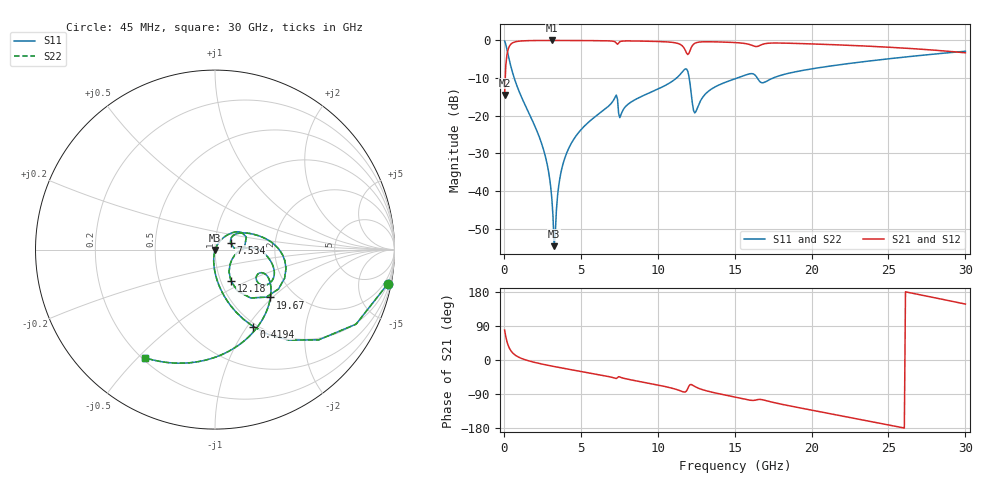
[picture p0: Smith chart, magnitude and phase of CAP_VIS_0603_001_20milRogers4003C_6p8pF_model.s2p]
! S-parameter model data by Modelithics Inc.  support@modelithics.com  813-866-6335  Tampa FL USA
! S-Parameter data specifications:
! Substrate: 20-mil Rogers 4003C, substrate thickness, H=0.508mm, Dielectric constant, Er=3.75
! PCB Mounting Pad Footprint: Pad width, PadW=0.90mm , Pad length, PadL=1.00mm , Pad gap, PadG (edge-to-edge)=1.00mm , Reference planes=3.0mm apart
! Created Wed Nov 18 13:24:22 2015
# hz S ma R 50
! 2 Port Network Data from SP1.SP block
! freq  magS11  angS11  magS21  angS21  magS12  angS12  magS22  angS22
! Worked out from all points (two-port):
!   401 points, 45 MHz to 30 GHz, reference 50 ohm
!   highest |S21| = -0.02 dB at 3.115 GHz (marker M1); lowest = -14.4 dB at 45 MHz (marker M2)
!   |S21| within 3 dB of the highest: 237.8 MHz to 11.84 GHz (11.6 GHz wide, 192 % of centre); 12.07 GHz to 29.26 GHz (17.19 GHz wide, 83.2 % of centre)
!   lowest |S11| = -54.6 dB at 3.265 GHz (marker M3), VSWR 1.00, Z = 50.1 - j0.145 ohm
!   |S11| at or under -10 dB: 671.1 MHz to 11.22 GHz (10.54 GHz wide, 177 % of centre); 12.04 GHz to 15.15 GHz (3.106 GHz wide, 22.8 % of centre); 16.48 GHz to 17.49 GHz (1.011 GHz wide, 5.96 % of centre)
!   |S22| runs from -54.6 to -0.2 dB; largest |S21 - S12| = 0
!   S11 on the Smith chart (normalised r, x): 45 MHz: 1, -10; 419.4 MHz: 0.96, -1.07; 7.534 GHz: 1.19, +0.09; 12.18 GHz: 1.12, -0.41; 19.67 GHz: 1.52, -0.97; 30 GHz: 0.21, -0.52
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4.5e7  0.9819 -11.2  0.1896 78.8  0.1896 78.8  0.9819 -11.2
4.194375e8  0.4796 -63.5  0.8769 26.4  0.8769 26.4  0.4796 -63.5
1.018538e9  0.2029 -83.4  0.9782 6.3  0.9782 6.3  0.2029 -83.4
2.591175e9  0.03463 -99.5  0.9978 -11.7  0.9978 -11.7  0.03463 -99.5
2.890725e9  0.01873 -99.8  0.9981 -14.2  0.9981 -14.2  0.01873 -99.8
3.115388e9  0.007989 -95.1  0.9982 -16.0  0.9982 -16.0  0.007989 -95.1
3.265162e9  0.001865 -51.0  0.9982 -17.2  0.9982 -17.2  0.001865 -51.0
3.93915e9  0.02673 63.9  0.9976 -22.4  0.9976 -22.4  0.02673 63.9
5.062462e9  0.06714 57.6  0.9953 -30.6  0.9953 -30.6  0.06714 57.6
7.2342e9  0.1775 32.0  0.954 -48.3  0.954 -48.3  0.1775 32.0
7.53375e9  0.09435 23.0  0.9599 -44.8  0.9599 -44.8  0.09435 23.0
1.007992e10  0.2301 21.9  0.9662 -66.6  0.9662 -66.6  0.2301 21.9
1.127812e10  0.3246 6.2  0.9155 -78.6  0.9155 -78.6  0.3246 6.2
1.180234e10  0.4194 -22.3  0.7306 -84.2  0.7306 -84.2  0.4194 -22.3
1.217678e10  0.1969 -63.2  0.8021 -64.8  0.8021 -64.8  0.1969 -63.2
1.247632e10  0.1133 -17.2  0.9283 -71.3  0.9283 -71.3  0.1133 -17.2
1.330009e10  0.2122 2.8  0.9596 -82.7  0.9596 -82.7  0.2122 2.8
1.50225e10  0.3096 -10.3  0.9361 -97.8  0.9361 -97.8  0.3096 -10.3
1.966552e10  0.408 -40.8  0.9028 -129.6  0.9028 -129.6  0.408 -40.8
2.003996e10  0.4202 -43.6  0.8976 -132.5  0.8976 -132.5  0.4202 -43.6
2.505742e10  0.5716 -82.3  0.8111 -171.7  0.8111 -171.7  0.5716 -82.3
3e10  0.718 -123.0  0.6845 147.6  0.6845 147.6  0.718 -123.0
